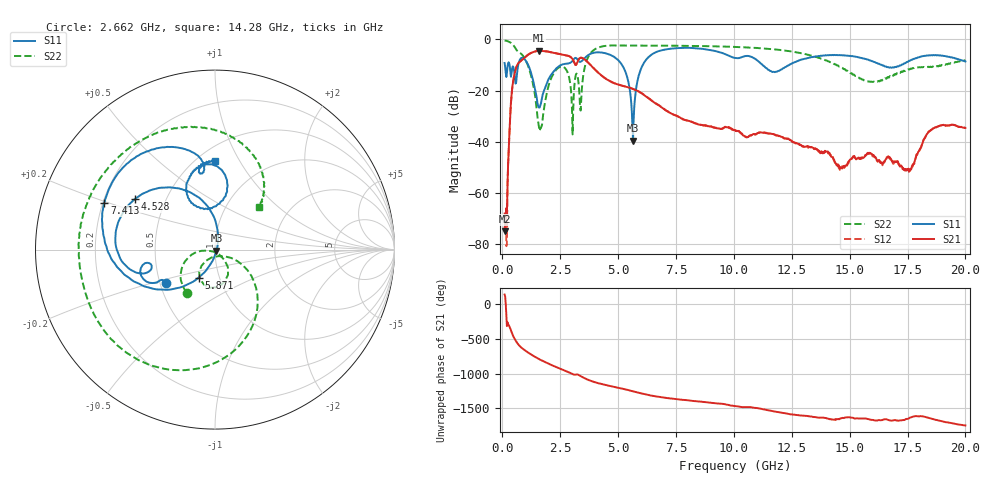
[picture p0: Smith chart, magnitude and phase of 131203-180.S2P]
!  2-Port S-parameters saved by WinCal
! VAR MeasName=S-Parameters (CALIBRATED_DATA) read from VNA (N5244A)
! VAR MeasDate=4/4/2013 3:59:52 PM
! VAR NAME=131203-180
! VAR FILENAME=131203-180.S2P
! VAR DATE=4/4/2013 3:59:52 PM
! VAR PHYS_PORTS=1,2
# Hz S MA R 50
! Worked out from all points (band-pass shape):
!   801 points, 100 MHz to 20 GHz, reference 50 ohm
!   highest |S21| = -4.42 dB at 1.568 GHz (marker M1); lowest = -75.2 dB at 124.9 MHz (marker M2)
!   |S21| within 3 dB of the highest: 927.2 MHz to 3.014 GHz (2.087 GHz wide, 106 % of centre); 3.333 GHz to 3.493 GHz (159.3 MHz wide, 4.67 % of centre)
!   lowest |S11| = -39.6 dB at 5.647 GHz (marker M3), VSWR 1.02, Z = 50.8 - j0.688 ohm
!   |S11| at or under -10 dB: 1.118 GHz to 2.54 GHz (1.422 GHz wide, 77.7 % of centre); 5.172 GHz to 6.065 GHz (893.2 MHz wide, 15.9 % of centre); 11.24 GHz to 12.39 GHz (1.143 GHz wide, 9.68 % of centre)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
!   |S22| runs from -37.2 to -0.4 dB; largest |S21 - S12| = 0.0022
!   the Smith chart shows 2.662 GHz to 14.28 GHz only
!   S11 on the Smith chart (normalised r, x): 2.662 GHz: 0.54, -0.23; 4.528 GHz: 0.33, +0.26; 5.871 GHz: 0.80, -0.26; 7.413 GHz: 0.21, +0.19; 14.28 GHz: 0.61, +0.80
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1e8  0.3465 153.0  0.0003867 143.8  0.0001845 -126.1  0.9575 -22.2
1.24875e8  0.2879 148.4  0.0001739 116.4  0.0003416 99.7  0.9535 -27.5
3.73625e8  0.1855 162.8  0.05708 -13.6  0.05745 -13.3  0.8572 -81.6
5.22875e8  0.2201 148.6  0.2052 -129.8  0.2059 -129.8  0.725 -112.6
9.4575e8  0.4219 142.3  0.4327 64.5  0.4334 64.5  0.4453 176.7
1.567625e9  0.04731 -10.3  0.6011 -65.7  0.6029 -65.7  0.02148 35.5
2.114875e9  0.2055 -115.3  0.5598 -153.9  0.5613 -153.9  0.1761 -45.7
2.662125e9  0.3297 -145.4  0.4987 130.0  0.5005 130.0  0.2855 -122.6
3.010375e9  0.3709 -150.4  0.428 78.0  0.4296 78.0  0.043 -172.6
3.43325e9  0.3778 -162.2  0.4366 35.7  0.438 35.6  0.1033 -27.1
3.756625e9  0.5083 -170.4  0.3349 -15.2  0.3355 -15.4  0.4949 -66.9
4.52775e9  0.5278 147.7  0.164 -88.4  0.1638 -88.5  0.7557 -129.5
5.274e9  0.2592 101.6  0.1211 -143.4  0.1213 -143.3  0.7618 -159.4
5.647125e9  0.01042 -40.5  0.1078 -174.7  0.108 -174.7  0.7595 -169.8
5.871e9  0.1803 -120.3  0.09663 166.0  0.09699 165.8  0.7596 -175.3
6.741625e9  0.5895 -177.4  0.05184 106.6  0.0521 106.2  0.7605 165.4
7.41325e9  0.6691 157.2  0.03325 76.4  0.03351 76.6  0.7551 152.8
1.005e10  0.4351 98.7  0.01659 -27.5  0.01638 -27.3  0.7153 109.9
1.338325e10  0.4529 105.9  0.007735 177.3  0.007587 177.9  0.4768 55.4
1.427875e10  0.4946 90.0  0.00483 137.5  0.005003 139.6  0.3426 43.6
1.669162e10  0.284 70.7  0.005064 128.3  0.004932 127.6  0.1788 95.9
2e10  0.3707 39.0  0.01855 51.9  0.01861 51.7  0.3934 94.0
